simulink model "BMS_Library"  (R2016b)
settings: Solver=VariableStepAuto  StartTime=0.0  StopTime=10.0  RelTol=1e-3
PreLoadFcn:
  | slblocks
  | sl_customization
undefined symbols (not defined in the file or in its folder): bin2dec
libraries: simulink x10

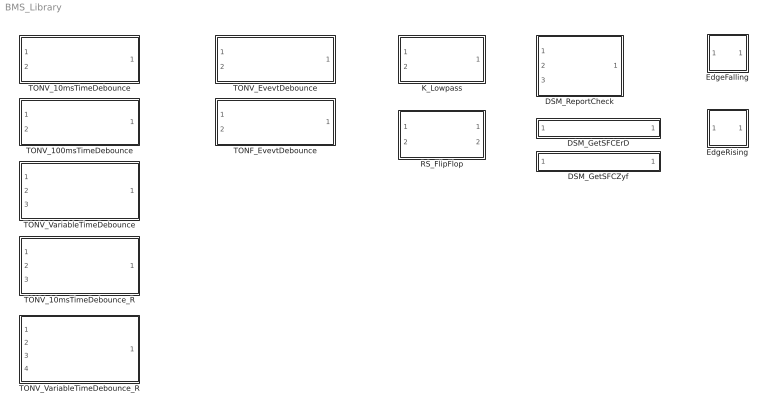
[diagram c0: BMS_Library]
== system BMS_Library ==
  DSM_GetSFCErD : Subsystem  TreatAsAtomicUnit=on  RTWFcnName=TONV_10msTimeDebounce  RTWFileName=SrvLib
  DSM_GetSFCZyf : Subsystem  TreatAsAtomicUnit=on  RTWFcnName=TONV_10msTimeDebounce  RTWFileName=SrvLib
  DSM_ReportCheck : Subsystem  TreatAsAtomicUnit=on  RTWFcnName=DSM_ReportCheck  RTWFileName=SrvLib
  EdgeFalling : Subsystem  TreatAsAtomicUnit=on  RTWFcnName=EdgeFalling  RTWFileName=SrvLib
  EdgeRising : Subsystem  TreatAsAtomicUnit=on  RTWFcnName=EdgeRising  RTWFileName=SrvLib
  K_Lowpass : Subsystem  TreatAsAtomicUnit=on  RTWFcnName=K_Lowpass  RTWFileName=SrvLib
  RS_FlipFlop : Subsystem
  TONF_EvevtDebounce : Subsystem  TreatAsAtomicUnit=on  RTWFcnName=TONF_EvevtDebounce  RTWFileName=SrvLib
  TONV_100msTimeDebounce : Subsystem  TreatAsAtomicUnit=on  RTWFcnName=TONV_100msTimeDebounce  RTWFileName=SrvLib
  TONV_10msTimeDebounce : Subsystem  TreatAsAtomicUnit=on  RTWFcnName=TONV_10msTimeDebounce  RTWFileName=SrvLib
  TONV_10msTimeDebounce_R : Subsystem  TreatAsAtomicUnit=on  RTWFcnName=TONV_10msTimeDebounce_R  RTWFileName=SrvLib
  TONV_EvevtDebounce : Subsystem  TreatAsAtomicUnit=on  RTWFcnName=TONV_EvevtDebounce  RTWFileName=SrvLib
  TONV_VariableTimeDebounce : Subsystem  TreatAsAtomicUnit=on  RTWFcnName=TONV_VariableTimeDebounce  RTWFileName=SrvLib
  TONV_VariableTimeDebounce_R : Subsystem  TreatAsAtomicUnit=on  RTWFcnName=TONV_VariableTimeDebounce_R  RTWFileName=SrvLib

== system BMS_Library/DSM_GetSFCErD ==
  DFC : Inport  OutDataTypeStr=uint8
  DFC_IsoChkLv1_1 : simulink/Logic and Bit Operations/Bitwise Operator  logicop=AND  UseBitMask=on  BitMask=bin2dec('00010000')  BitMaskRealWorld=Stored Integer
  DFC_IsoChkLv1_1_compare : simulink/Logic and Bit Operations/Compare To Constant  relop===  const=16  OutDataTypeStr=boolean
  y : Outport
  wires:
  DFC_IsoChkLv1_1_compare/1 -> y/1
  DFC/1 -> DFC_IsoChkLv1_1/1
  DFC_IsoChkLv1_1/1 -> DFC_IsoChkLv1_1_compare/1

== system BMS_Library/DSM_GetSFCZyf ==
  DFC : Inport  OutDataTypeStr=uint8
  DFC_IsoChkLv1_1 : simulink/Logic and Bit Operations/Bitwise Operator  logicop=AND  UseBitMask=on  BitMask=bin2dec('00001000')  BitMaskRealWorld=Stored Integer
  DFC_IsoChkLv1_1_compare1 : simulink/Logic and Bit Operations/Compare To Constant  relop===  const=8  OutDataTypeStr=boolean
  y : Outport
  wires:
  DFC_IsoChkLv1_1_compare1/1 -> y/1
  DFC/1 -> DFC_IsoChkLv1_1/1
  DFC_IsoChkLv1_1/1 -> DFC_IsoChkLv1_1_compare1/1

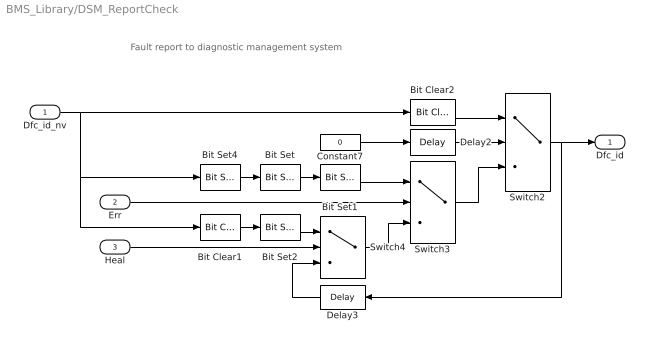
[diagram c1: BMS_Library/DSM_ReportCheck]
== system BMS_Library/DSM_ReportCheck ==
  note: Fault report to diagnostic management system
  Dfc_id_nv : Inport  OutDataTypeStr=uint8
  Err : Inport  Port=2
  Heal : Inport  Port=3
  Bit Clear1 : simulink/Logic and Bit Operations/Bit Clear  iBit=4
  Bit Clear2 : simulink/Logic and Bit Operations/Bit Clear  iBit=3
  Bit Set : simulink/Logic and Bit Operations/Bit Set  iBit=4
  Bit Set1 : simulink/Logic and Bit Operations/Bit Set  iBit=3
  Bit Set2 : simulink/Logic and Bit Operations/Bit Set  iBit=3
  Bit Set4 : simulink/Logic and Bit Operations/Bit Set  iBit=7
  Constant7 : Constant  Value=0  OutDataTypeStr=boolean
  Delay2 : Delay  DelayLength=1  InitialCondition=1
  Delay3 : Delay  DelayLength=1  InitialCondition=0
  Switch2 : Switch  Criteria=u2 ~= 0
  Switch3 : Switch  Criteria=u2 ~= 0
  Switch4 : Switch  Criteria=u2 ~= 0
  Dfc_id : Outport  OutDataTypeStr=uint8
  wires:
  Heal/1 -> Switch4/2
  Delay3/1 -> Switch4/3
  Bit Clear1/1 -> Bit Set2/1
  Bit Set2/1 -> Switch4/1
  Err/1 -> Switch3/2
  Switch4/1 -> Switch3/3
  Bit Set/1 -> Bit Set1/1
  Bit Set1/1 -> Switch3/1
  Switch2/1 -> Dfc_id/1, Delay3/1
  Bit Clear2/1 -> Switch2/1
  Switch3/1 -> Switch2/3
  Delay2/1 -> Switch2/2
  Constant7/1 -> Delay2/1
  Bit Set4/1 -> Bit Set/1
  Dfc_id_nv/1 -> Bit Clear1/1, Bit Set4/1, Bit Clear2/1

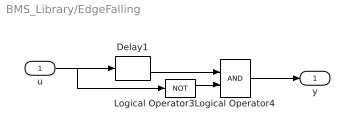
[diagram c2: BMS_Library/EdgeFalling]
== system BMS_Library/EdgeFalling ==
  u : Inport
  Delay1 : Delay  DelayLength=1  InitialCondition=0
  Logical Operator3 : Logic  Operator=NOT  AllPortsSameDT=off  OutDataTypeStr=boolean
  Logical Operator4 : Logic  AllPortsSameDT=off  OutDataTypeStr=boolean
  y : Outport
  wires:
  Logical Operator4/1 -> y/1
  u/1 -> Delay1/1, Logical Operator3/1
  Logical Operator3/1 -> Logical Operator4/2
  Delay1/1 -> Logical Operator4/1

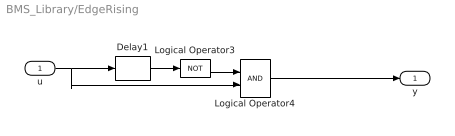
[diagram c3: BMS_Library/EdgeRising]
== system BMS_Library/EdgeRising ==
  u : Inport
  Delay1 : Delay  DelayLength=1  InitialCondition=1
  Logical Operator3 : Logic  Operator=NOT  AllPortsSameDT=off  OutDataTypeStr=boolean
  Logical Operator4 : Logic  AllPortsSameDT=off  OutDataTypeStr=boolean
  y : Outport
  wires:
  Delay1/1 -> Logical Operator3/1
  u/1 -> Logical Operator4/2, Delay1/1
  Logical Operator3/1 -> Logical Operator4/1
  Logical Operator4/1 -> y/1

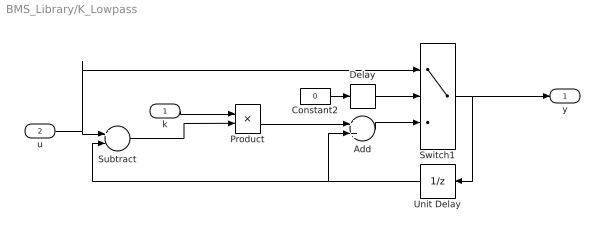
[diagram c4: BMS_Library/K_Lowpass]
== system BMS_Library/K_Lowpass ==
  k : Inport
  u : Inport  Port=2
  Add : Sum
  Constant2 : Constant  Value=0
  Delay : Delay  DelayLength=1  InitialCondition=1
  Product : Product
  Subtract : Sum  Inputs=+-
  Switch1 : Switch  Criteria=u2 > Threshold
  Unit Delay : UnitDelay  SampleTime=-1
  y : Outport
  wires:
  k/1 -> Product/1
  Product/1 -> Add/1
  Constant2/1 -> Delay/1
  Unit Delay/1 -> Subtract/2, Add/2
  Subtract/1 -> Product/2
  Add/1 -> Switch1/3
  Delay/1 -> Switch1/2
  Switch1/1 -> y/1, Unit Delay/1
  u/1 -> Switch1/1, Subtract/1

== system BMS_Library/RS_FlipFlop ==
  S : Inport  OutDataTypeStr=boolean
  R : Inport  Port=2  OutDataTypeStr=boolean
  RS : Stateflow chart  TreatAsAtomicUnit=on
  Q : Outport  OutDataTypeStr=boolean
  !Q : Outport  Port=2  OutDataTypeStr=boolean
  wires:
  RS/1(Q) -> Q/1
  RS/2(nQ) -> !Q/1
  S/1 -> RS/1(S)
  R/1 -> RS/2(R)

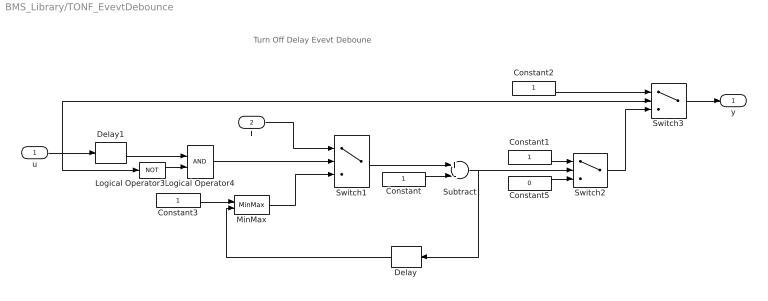
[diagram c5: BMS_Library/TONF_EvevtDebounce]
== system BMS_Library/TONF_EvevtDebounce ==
  note: Turn Off Delay Evevt Deboune
  u : Inport
  T : Inport  Port=2
  Constant : Constant  OutDataTypeStr=uint8
  Constant1 : Constant  OutDataTypeStr=boolean
  Constant2 : Constant  OutDataTypeStr=boolean
  Constant3 : Constant  OutDataTypeStr=single
  Constant5 : Constant  Value=0  OutDataTypeStr=boolean
  Delay : Delay  DelayLength=1  InitialCondition=0
  Delay1 : Delay  DelayLength=1  InitialCondition=0
  Logical Operator3 : Logic  Operator=NOT  AllPortsSameDT=off  OutDataTypeStr=boolean
  Logical Operator4 : Logic  AllPortsSameDT=off  OutDataTypeStr=boolean
  MinMax : MinMax  Function=max  Inputs=2
  Subtract : Sum  Inputs=+-  OutDataTypeStr=single
  Switch1 : Switch  Criteria=u2 > Threshold
  Switch2 : Switch  Criteria=u2 > Threshold
  Switch3 : Switch  Criteria=u2 > Threshold
  y : Outport
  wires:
  Constant1/1 -> Switch2/1
  Constant5/1 -> Switch2/3
  u/1 -> Switch3/2, Delay1/1, Logical Operator3/1
  Delay1/1 -> Logical Operator4/1
  Logical Operator3/1 -> Logical Operator4/2
  Logical Operator4/1 -> Switch1/2
  Delay/1 -> MinMax/2
  T/1 -> Switch1/1
  Switch1/1 -> Subtract/1
  Subtract/1 -> Switch2/2, Delay/1
  Constant/1 -> Subtract/2
  Constant3/1 -> MinMax/1
  MinMax/1 -> Switch1/3
  Switch2/1 -> Switch3/3
  Constant2/1 -> Switch3/1
  Switch3/1 -> y/1

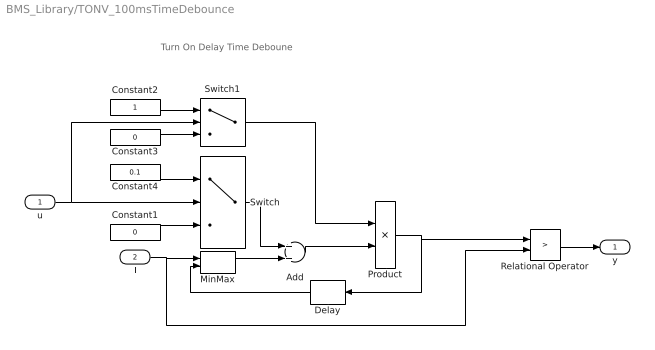
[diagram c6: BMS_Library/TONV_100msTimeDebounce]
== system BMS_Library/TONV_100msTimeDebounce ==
  note: Turn On Delay Time Deboune
  u : Inport
  T : Inport  Port=2
  Add : Sum
  Constant1 : Constant  Value=0  OutDataTypeStr=single
  Constant2 : Constant  OutDataTypeStr=uint8
  Constant3 : Constant  Value=0  OutDataTypeStr=uint8
  Constant4 : Constant  Value=0.1  OutDataTypeStr=single
  Delay : Delay  DelayLength=1  InitialCondition=0
  MinMax : MinMax  Inputs=2
  Product : Product  OutMin=[0]  OutMax=[65535]  OutDataTypeStr=single
  Relational Operator : RelationalOperator  Operator=>  OutDataTypeStr=boolean  RndMeth=Simplest
  Switch : Switch  Criteria=u2 ~= 0
  Switch1 : Switch  Criteria=u2 ~= 0
  y : Outport
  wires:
  MinMax/1 -> Add/2
  T/1 -> Relational Operator/2, MinMax/1
  Relational Operator/1 -> y/1
  Delay/1 -> MinMax/2
  Switch/1 -> Add/1
  Product/1 -> Delay/1, Relational Operator/1
  Add/1 -> Product/2
  Constant1/1 -> Switch/3
  Constant4/1 -> Switch/1
  u/1 -> Switch/2, Switch1/2
  Constant2/1 -> Switch1/1
  Constant3/1 -> Switch1/3
  Switch1/1 -> Product/1

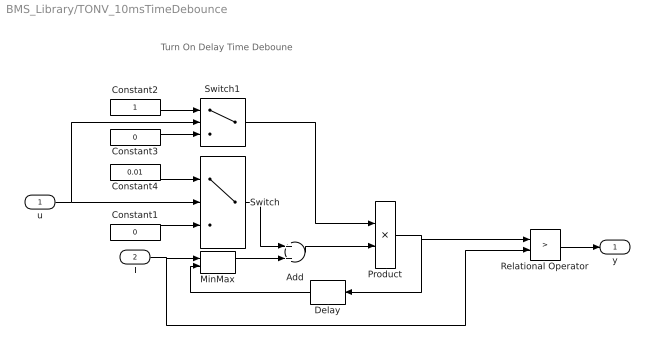
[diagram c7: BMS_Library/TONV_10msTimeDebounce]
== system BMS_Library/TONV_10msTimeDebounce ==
  note: Turn On Delay Time Deboune
  u : Inport
  T : Inport  Port=2
  Add : Sum
  Constant1 : Constant  Value=0  OutDataTypeStr=single
  Constant2 : Constant  OutDataTypeStr=uint8
  Constant3 : Constant  Value=0  OutDataTypeStr=uint8
  Constant4 : Constant  Value=0.01  OutDataTypeStr=single
  Delay : Delay  DelayLength=1  InitialCondition=0
  MinMax : MinMax  Inputs=2
  Product : Product  OutMin=[0]  OutMax=[65535]  OutDataTypeStr=single
  Relational Operator : RelationalOperator  Operator=>  OutDataTypeStr=boolean  RndMeth=Simplest
  Switch : Switch  Criteria=u2 ~= 0
  Switch1 : Switch  Criteria=u2 ~= 0
  y : Outport
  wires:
  Switch1/1 -> Product/1
  Constant3/1 -> Switch1/3
  Constant2/1 -> Switch1/1
  u/1 -> Switch1/2, Switch/2
  Constant4/1 -> Switch/1
  Constant1/1 -> Switch/3
  Add/1 -> Product/2
  Product/1 -> Relational Operator/1, Delay/1
  Switch/1 -> Add/1
  Delay/1 -> MinMax/2
  Relational Operator/1 -> y/1
  T/1 -> MinMax/1, Relational Operator/2
  MinMax/1 -> Add/2

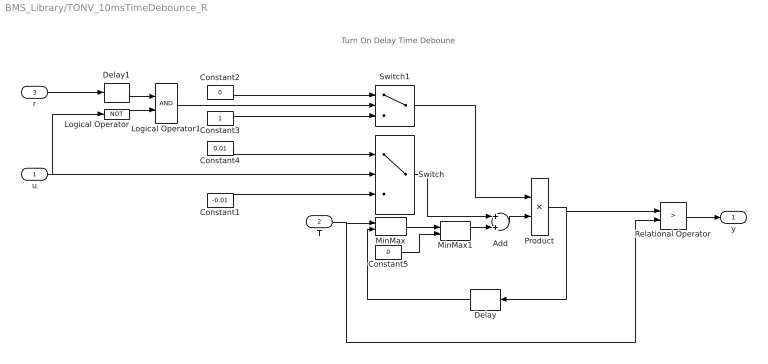
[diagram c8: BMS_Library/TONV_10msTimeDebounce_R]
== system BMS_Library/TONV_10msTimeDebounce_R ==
  note: Turn On Delay Time Deboune
  u : Inport
  T : Inport  Port=2
  r : Inport  Port=3
  Add : Sum
  Constant1 : Constant  Value=-0.01  OutDataTypeStr=single
  Constant2 : Constant  Value=0  OutDataTypeStr=uint8
  Constant3 : Constant  OutDataTypeStr=uint8
  Constant4 : Constant  Value=0.01  OutDataTypeStr=single
  Constant5 : Constant  Value=0  OutDataTypeStr=uint8
  Delay : Delay  DelayLength=1  InitialCondition=0
  Delay1 : Delay  DelayLength=1  InitialCondition=0
  Logical Operator : Logic  Operator=NOT  AllPortsSameDT=off  OutDataTypeStr=boolean
  Logical Operator1 : Logic  AllPortsSameDT=off  OutDataTypeStr=boolean
  MinMax : MinMax  Inputs=2
  MinMax1 : MinMax  Function=max  Inputs=2
  Product : Product  OutMin=[0]  OutMax=[65535]  OutDataTypeStr=single
  Relational Operator : RelationalOperator  Operator=>  OutDataTypeStr=boolean  RndMeth=Simplest
  Switch : Switch  Criteria=u2 ~= 0
  Switch1 : Switch  Criteria=u2 > Threshold
  y : Outport
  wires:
  Constant5/1 -> MinMax1/2
  MinMax1/1 -> Add/2
  Logical Operator1/1 -> Switch1/2
  Logical Operator/1 -> Logical Operator1/2
  Delay1/1 -> Logical Operator1/1
  r/1 -> Delay1/1
  Constant1/1 -> Switch/3
  MinMax/1 -> MinMax1/1
  T/1 -> Relational Operator/2, MinMax/1
  Relational Operator/1 -> y/1
  Delay/1 -> MinMax/2
  Switch/1 -> Add/1
  Product/1 -> Delay/1, Relational Operator/1
  Add/1 -> Product/2
  Constant4/1 -> Switch/1
  u/1 -> Logical Operator/1, Switch/2
  Constant2/1 -> Switch1/1
  Constant3/1 -> Switch1/3
  Switch1/1 -> Product/1

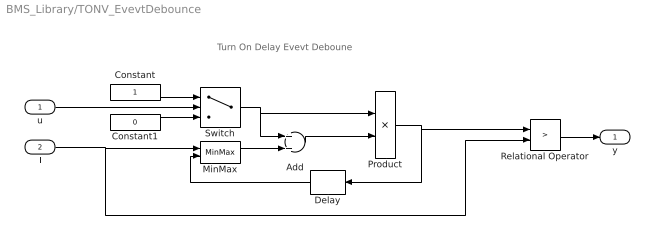
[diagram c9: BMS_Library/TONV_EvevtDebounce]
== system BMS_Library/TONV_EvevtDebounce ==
  note: Turn On Delay Evevt Deboune
  u : Inport
  T : Inport  Port=2
  Add : Sum
  Constant : Constant  OutDataTypeStr=uint8
  Constant1 : Constant  Value=0  OutDataTypeStr=uint8
  Delay : Delay  DelayLength=1  InitialCondition=0
  MinMax : MinMax  Inputs=2
  Product : Product  OutMin=[0]  OutMax=[65535]  OutDataTypeStr=single
  Relational Operator : RelationalOperator  Operator=>  OutDataTypeStr=boolean  RndMeth=Simplest
  Switch : Switch  Criteria=u2 > Threshold
  y : Outport
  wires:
  u/1 -> Switch/2
  Constant/1 -> Switch/1
  Constant1/1 -> Switch/3
  Add/1 -> Product/2
  Product/1 -> Relational Operator/1, Delay/1
  Switch/1 -> Add/1, Product/1
  Delay/1 -> MinMax/2
  Relational Operator/1 -> y/1
  T/1 -> Relational Operator/2, MinMax/1
  MinMax/1 -> Add/2

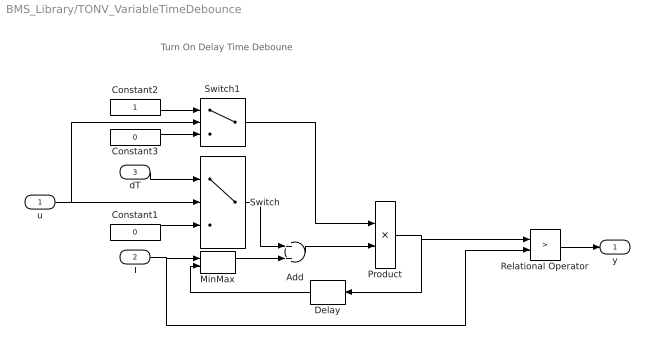
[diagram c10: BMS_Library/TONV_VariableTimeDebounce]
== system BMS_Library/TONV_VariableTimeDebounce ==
  note: Turn On Delay Time Deboune
  u : Inport
  T : Inport  Port=2
  dT : Inport  Port=3
  Add : Sum
  Constant1 : Constant  Value=0  OutDataTypeStr=single
  Constant2 : Constant  OutDataTypeStr=uint8
  Constant3 : Constant  Value=0  OutDataTypeStr=uint8
  Delay : Delay  DelayLength=1  InitialCondition=0
  MinMax : MinMax  Inputs=2
  Product : Product  OutMin=[0]  OutMax=[65535]  OutDataTypeStr=single
  Relational Operator : RelationalOperator  Operator=>  OutDataTypeStr=boolean  RndMeth=Simplest
  Switch : Switch  Criteria=u2 ~= 0
  Switch1 : Switch  Criteria=u2 ~= 0
  y : Outport
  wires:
  MinMax/1 -> Add/2
  T/1 -> Relational Operator/2, MinMax/1
  Relational Operator/1 -> y/1
  Delay/1 -> MinMax/2
  Switch/1 -> Add/1
  Product/1 -> Delay/1, Relational Operator/1
  Add/1 -> Product/2
  Constant1/1 -> Switch/3
  dT/1 -> Switch/1
  u/1 -> Switch/2, Switch1/2
  Constant2/1 -> Switch1/1
  Constant3/1 -> Switch1/3
  Switch1/1 -> Product/1

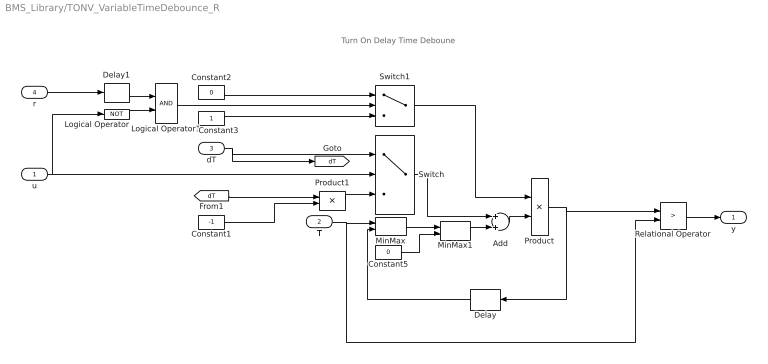
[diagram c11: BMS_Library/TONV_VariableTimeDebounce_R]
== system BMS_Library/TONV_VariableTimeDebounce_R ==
  note: Turn On Delay Time Deboune
  u : Inport
  T : Inport  Port=2
  dT : Inport  Port=3
  r : Inport  Port=4
  Add : Sum
  Constant1 : Constant  Value=-1  OutDataTypeStr=single
  Constant2 : Constant  Value=0  OutDataTypeStr=uint8
  Constant3 : Constant  OutDataTypeStr=uint8
  Constant5 : Constant  Value=0  OutDataTypeStr=uint8
  Delay : Delay  DelayLength=1  InitialCondition=0
  Delay1 : Delay  DelayLength=1  InitialCondition=0
  Logical Operator : Logic  Operator=NOT  AllPortsSameDT=off  OutDataTypeStr=boolean
  Logical Operator1 : Logic  AllPortsSameDT=off  OutDataTypeStr=boolean
  MinMax : MinMax  Inputs=2
  MinMax1 : MinMax  Function=max  Inputs=2
  Product : Product  OutMin=[0]  OutMax=[65535]  OutDataTypeStr=single
  Product1 : Product
  Relational Operator : RelationalOperator  Operator=>  OutDataTypeStr=boolean  RndMeth=Simplest
  Switch : Switch  Criteria=u2 ~= 0
  Switch1 : Switch  Criteria=u2 > Threshold
  y : Outport
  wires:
  Switch1/1 -> Product/1
  Constant3/1 -> Switch1/3
  Constant2/1 -> Switch1/1
  u/1 -> Switch/2, Logical Operator/1
  dT/1 -> Switch/1, [dT]
  Add/1 -> Product/2
  Product/1 -> Relational Operator/1, Delay/1
  Switch/1 -> Add/1
  Delay/1 -> MinMax/2
  Relational Operator/1 -> y/1
  T/1 -> MinMax/1, Relational Operator/2
  MinMax/1 -> MinMax1/1
  Constant1/1 -> Product1/2
  Product1/1 -> Switch/3
  [dT] -> Product1/1
  r/1 -> Delay1/1
  Delay1/1 -> Logical Operator1/1
  Logical Operator/1 -> Logical Operator1/2
  Logical Operator1/1 -> Switch1/2
  MinMax1/1 -> Add/2
  Constant5/1 -> MinMax1/2

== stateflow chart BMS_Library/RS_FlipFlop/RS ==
  state RS_FlipFlop
    (default) -> (junction 3)
    (junction 3) -> (junction 5) : [R]
    (junction 3) -> (junction 12)
    (junction 5) -> (junction 7) : {Q=boolean(0);nQ=boolean(1);}
    (junction 12) -> (junction 14) : [S]
    (junction 14) -> (junction 16) : {Q=boolean(1);nQ=boolean(0);}
    (junction 12) -> (junction 18)
    (junction 16) -> (junction 18)
    (junction 7) -> (junction 18)
    (junction 18) -> (junction 21)
  (default) -> RS_FlipFlop
  (junction 24) -> RS_FlipFlop
  (junction 25) -> (junction 24)
  RS_FlipFlop -> (junction 23)
  (junction 23) -> (junction 25)
  data: S input boolean; R input boolean; Q output boolean; nQ output boolean
